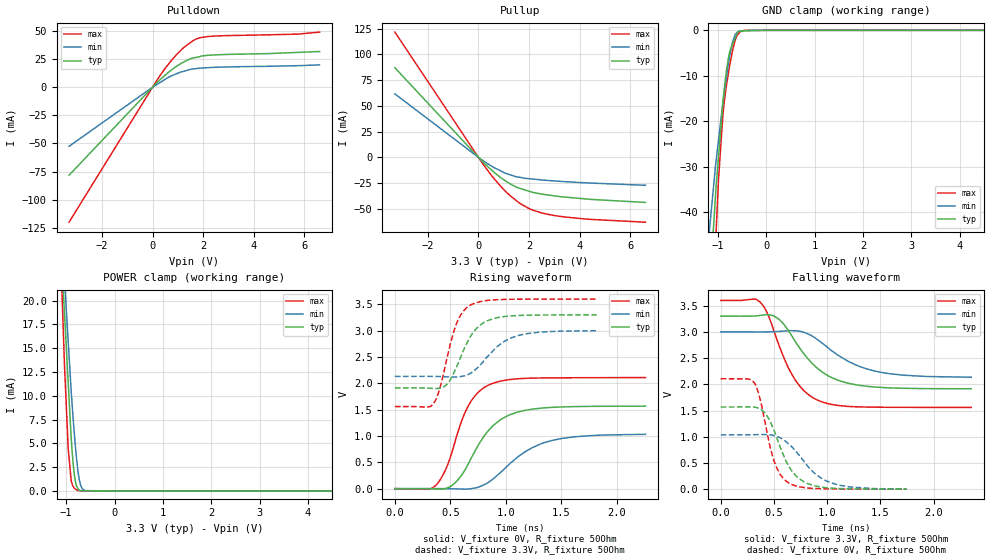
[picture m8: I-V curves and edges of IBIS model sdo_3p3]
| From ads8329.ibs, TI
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|   sdo_3p3 Model
[Model]   sdo_3p3
Model_type   3-state
Polarity   Non-Inverting
Vmeas = 1.65
Vref = 1.65
Cref = 30pF
Rref = 50
|   typ   min   max
|   (nom PVT)   (Fast PVT)   (slow PVT)
|C_comp from frequency sweep method(F=0.05MHz)
|C_comp   7.932e-12   5.196e-12   1.737e-11
|ON state : BUFFER OUTPUT TURNED HIGH
|C_comp   7.932e-12   5.196e-12   1.737e-11
|OFF state: BUFFER IN HIGH IMPEDANCE
|C_comp   3.907e-12   4.055e-12   3.753e-12
|C_comp from LC tank measurement(L=1nH)
C_comp   3.031e-12   2.7275e-12  3.2545e-12
|OFF state: BUFFER IN HIGH IMPEDANCE
|Resonant Frequency(Hz)   2.970e+09   3.100e+09   2.880e+09
|C_comp   2.874e-12   2.638e-12   3.057e-12
|ON state : BUFFER OUTPUT TURNED HIGH
|Resonant Frequency(Hz)   2.820e+09   3.000e+09   2.710e+09
|C_comp   3.188e-12   2.817e-12   3.452e-12
| Where nom  PVT is Nominal Process,  3.3V,  28C
|   Fast PVT is Strong Process,   3.6V,  -40C
|   Slow PVT is Weak Process,   3V,  88C
[Voltage Range]   3.3   3   3.6
|Ambient Temperature   25   85   -40
|Junction Temperature
[Temperature Range]   28   88   -40
[Pullup Reference]   3.3   3   3.6
[Pulldown Reference]   0   0   0
[Power Clamp Reference]   3.3   3   3.6
[GND Clamp Reference]   0   0   0
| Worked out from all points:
|   slope of the pulldown table from 0 to 0.495 V, typ, clamps not added: 46.5 ohm
|   slope of the pullup table from 0 to 0.495 V, typ, clamps not added: 41.8 ohm
|   GND clamp passes 1 mA (typ) near -0.61 V on its own axis
|   POWER clamp passes 1 mA (typ) near -0.81 V on its own axis
|   falling waveform, V_fixture 3.3V, R_fixture 50Ohm: 20-80 % time 348ps typ, 425ps min, 272ps max; typ from 3.3 V to 1.92 V
|   rising waveform, V_fixture 0V, R_fixture 50Ohm: 20-80 % time 298ps typ, 391ps min, 226ps max; typ from 0 V to 1.56 V
|   rising waveform, V_fixture 3.3V, R_fixture 50Ohm: 20-80 % time 198ps typ, 263ps min, 154ps max; typ from 1.91 V to 3.3 V
|   falling waveform, V_fixture 0V, R_fixture 50Ohm: 20-80 % time 209ps typ, 288ps min, 149ps max; typ from 1.57 V to 0.003 V
[Pulldown]
|   Voltage   I(typ)   I(min)   I(max)
-3.3V     -78.31mA   -52.56mA   -120.1mA
172.8mV   4.001mA    2.441mA    6.177mA
478.8mV   10.34mA    6.702mA    16.15mA
770.4mV   15.77mA    10.32mA    24.48mA
1.246V    22.65mA    14.27mA    35.48mA
1.554V    25.79mA    16.09mA    40.64mA
1.706V    26.43mA    16.53mA    42.69mA
2.167V    28.35mA    17.37mA    45.04mA
5.778V    31.01mA    19.17mA    47.29mA
6.6V      31.76mA    19.87mA    49.04mA
[GND Clamp]
|   Voltage   I(typ)   I(min)   I(max)
-3.3V     -511.9mA   -370.7mA   -746.5mA
-1.204V   -62.26mA   -47.41mA   -87.55mA
-1.102V   -45.26mA   -35.81mA   -59.55mA
-1.033V   -33.91mA   -28.37mA   -43.59mA
-986.4mV  -27.74mA   -24.15mA   -32.78mA
-896.4mV  -15.82mA   -16mA      -18.72mA
-860.4mV  -12.18mA   -13.11mA   -15.1mA
-782.1mV  -6.131mA   -7.349mA   -9.442mA
-705mV    -3.276mA   -2.926mA   -4.937mA
-608.4mV  -871.8uA   -542.8uA   -1.177mA
-549mV    -198.7uA   -140.8uA   -475.7uA
6.6V      0A         0A         0A
[Pullup]
|   Voltage   I(typ)   I(min)   I(max)
-3.3V     86.97mA    61.59mA    121.7mA
234mV     -5.884mA   -4.117mA   -8.357mA
604.8mV   -14.26mA   -9.827mA   -20.34mA
939.6mV   -20.77mA   -13.98mA   -29.76mA
1.246V    -25.69mA   -16.95mA   -37.13mA
1.609V    -30.02mA   -19.39mA   -44.24mA
2.167V    -34.22mA   -21.23mA   -51.5mA
2.624V    -36.23mA   -22.29mA   -54.8mA
3.089V    -37.81mA   -23.15mA   -56.94mA
4.497V    -41.02mA   -25.13mA   -60.46mA
6.6V      -43.88mA   -27.24mA   -63.09mA
[POWER Clamp]
|   Voltage   I(typ)   I(min)   I(max)
-3.3V     177.2mA    159.5mA    202.3mA
-1.451V   64.21mA    57.65mA    74.35mA
-1.053V   20.33mA    23.75mA    15.75mA
-1.033V   18.48mA    22.09mA    12.93mA
-957.6mV  11.32mA    15.65mA    4.394mA
-896.4mV  5.55mA     10.45mA    1.07mA
-858mV    2.977mA    7.726mA    487.3uA
-825mV    1.439mA    5.582mA    239.7uA
-756mV    230.5uA    2.053mA    40.29uA
-696mV    31.36uA    516.1uA    6.841uA
-591mV    26.61uA    22.96uA    1.622uA
6.6V      0A         0A         0A
[Ramp]
R_load = 50
|   typ   min   max
dV/dt_r   0.940692/2.96669e-10   0.62254/3.92244e-10   1.26583/2.26055e-10
dV/dt_f   0.831733/3.49421e-10   0.521048/4.29466e-10   1.22475/2.7179e-10
[Falling Waveform]
V_fixture = 3.3V
V_fixture_min = 3V
V_fixture_max = 3.6V
R_fixture = 50Ohm
|   Time   V(typ)   V(min)   V(max)
0s        3.3V       3V         3.6V
374ps     3.315V     2.999V     3.56V
430ps     3.329V     3V         3.389V
506ps     3.296V     3.005V     2.979V
660ps     2.949V     3.024V     2.219V
782ps     2.58V      2.992V     1.879V
924ps     2.28V      2.829V     1.687V
1.114ns   2.07V      2.539V     1.595V
1.42ns    1.954V     2.267V     1.566V
2.352ns   1.916V     2.136V     1.56V
[Rising Waveform]
V_fixture = 0V
V_fixture_min = 0V
V_fixture_max = 0V
R_fixture = 50Ohm
|   Time   V(typ)   V(min)   V(max)
0s        1.203nV    1.361nV    1.013nV
374ps     -6.593mV   536.9uV    72.85mV
452ps     615uV      -291.1uV   340.3mV
526ps     81mV       -3.15mV    775.5mV
660ps     464.9mV    -6.818mV   1.567V
754ps     836.7mV    30.09mV    1.835V
868ps     1.162V     157.3mV    1.989V
1.032ns   1.4V       469mV      2.07V
1.372ns   1.537V     890.2mV    2.102V
2.256ns   1.565V     1.032V     2.108V
[Rising Waveform]
V_fixture = 3.3V
V_fixture_min = 3V
V_fixture_max = 3.6V
R_fixture = 50Ohm
|   Time   V(typ)   V(min)   V(max)
0s        1.913V     2.131V     1.558V
348ps     1.901V     2.131V     1.617V
402ps     1.905V     2.128V     1.885V
462ps     1.969V     2.123V     2.409V
554ps     2.304V     2.119V     3.128V
612ps     2.601V     2.135V     3.357V
684ps     2.9V       2.194V     3.488V
848ps     3.2V       2.538V     3.576V
1.108ns   3.286V     2.905V     3.595V
1.818ns   3.298V     2.998V     3.598V
[Falling Waveform]
V_fixture = 0V
V_fixture_min = 0V
V_fixture_max = 0V
R_fixture = 50Ohm
|   Time   V(typ)   V(min)   V(max)
0s        1.568V     1.039V     2.108V
320ps     1.565V     1.041V     2.017V
364ps     1.541V     1.044V     1.764V
426ps     1.427V     1.043V     1.177V
504ps     1.106V     1.022V     523.7mV
566ps     767.7mV    972.9mV    263.5mV
642ps     430.2mV    859.3mV    118.5mV
786ps     137.9mV    522.9mV    32.41mV
992ps     30.92mV    159.1mV    9.945mV
1.744ns   3.466mV    4.578mV    3.155mV
